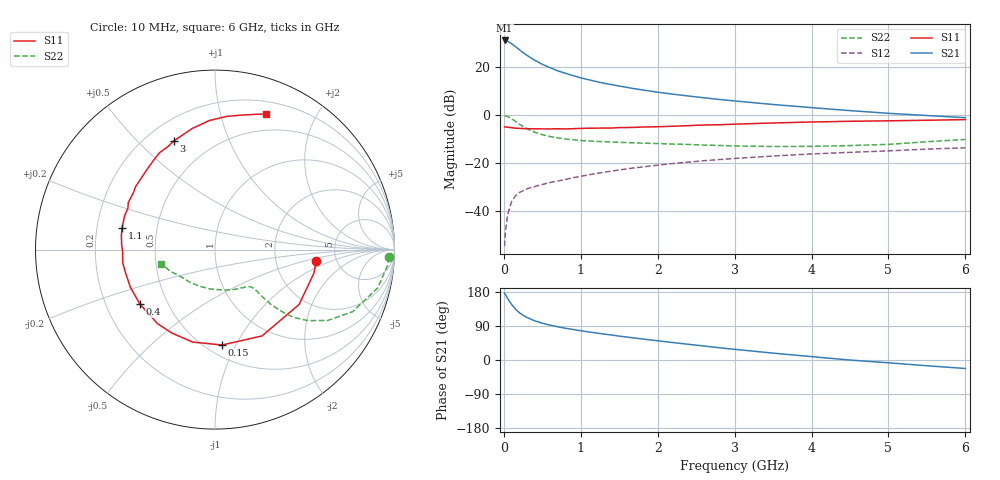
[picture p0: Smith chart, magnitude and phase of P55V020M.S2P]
! SIEMENS Small Signal Semiconductors
! BFP183
! Si NPN RF Bipolar Junction Transistor in SOT143
! VCE = 5 V  IC = 20 mA
! Common Emitter S-Parameters:  March  1996
# GHz  S  MA  R  50
!  f  S11  S21  S12  S22
! GHz  MAG  ANG  MAG  ANG  MAG  ANG  MAG  ANG
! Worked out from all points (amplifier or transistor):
!   36 points, 10 MHz to 6 GHz, reference 50 ohm
!   highest |S21| = 31.3 dB at 10 MHz (marker M1)
!   |S21| within 3 dB of that: start of sweep to 168 MHz
!   unconditionally stable (mu >= 1): 876.4 MHz to 5.61 GHz
!   at 250 MHz: K = 0.47, MSG = 28.9 dB, |S12| = -31.7 dB
!   at 1.4 GHz: K = 1.13, MAG = 16.0 dB, |S12| = -23.5 dB
!   at 6 GHz: K = 0.95, MSG = 6.3 dB, |S12| = -13.7 dB
!   S11 on the Smith chart (normalised r, x): 10 MHz: 3.48, -0.68; 150 MHz: 0.59, -0.88; 400 MHz: 0.35, -0.29; 1.1 GHz: 0.31, +0.11; 3 GHz: 0.31, +0.65; 6 GHz: 0.32, +1.39
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0.01  0.5677 -6.7  36.76 176.1  0.0018 87.7  0.9692 -2.5
0.02  0.5664 -13.5  36.68 172.8  0.0036 85.3  0.9646 -5.4
0.05  0.5594 -33.1  35.51 162.0  0.0084 79.3  0.9316 -13.2
0.1  0.5477 -61.4  31.43 146.9  0.0153 65.4  0.8408 -24.3
0.15  0.533 -85.7  27.44 134.4  0.0203 58.4  0.7415 -32.2
0.2  0.5301 -103.5  23.7 125.1  0.0239 54.1  0.6515 -37.4
0.25  0.5236 -117.1  20.41 117.9  0.026 51.1  0.5796 -40.7
0.3  0.5221 -127.8  17.97 112.4  0.0287 50.1  0.5207 -42.5
0.4  0.517 -144.1  14.22 103.4  0.0319 48.4  0.4407 -44.4
0.5  0.516 -155.9  11.62 97.1  0.0353 48.5  0.3895 -44.8
0.6  0.5148 -164.7  9.907 92.0  0.0389 49.2  0.3565 -44.9
0.7  0.5194 -171.9  8.505 87.7  0.0417 50.3  0.3333 -44.8
0.9  0.5213 176.6  6.738 80.6  0.049 51.6  0.3048 -45.1
1.1  0.532 166.7  5.543 74.0  0.0563 52.3  0.2877 -46.2
1.5  0.5493 151.6  4.073 63.0  0.0714 51.9  0.2697 -50.4
1.8  0.5646 141.8  3.386 55.4  0.082 50.9  0.259 -55.3
2.2  0.5858 130.2  2.754 45.9  0.0972 48.0  0.248 -62.8
3  0.6477 110.6  1.988 28.2  0.1239 41.5  0.2263 -82.4
3.5  0.6862 100.8  1.673 18.1  0.1394 37.2  0.2207 -97.0
4.5  0.7445 85.1  1.246 -0.1  0.1664 28.2  0.2306 -129.2
5.5  0.7823 74.2  0.983 -15.2  0.1946 20.6  0.2777 -154.4
6  0.8075 69.4  0.886 -22.4  0.2071 16.0  0.3098 -165.3
